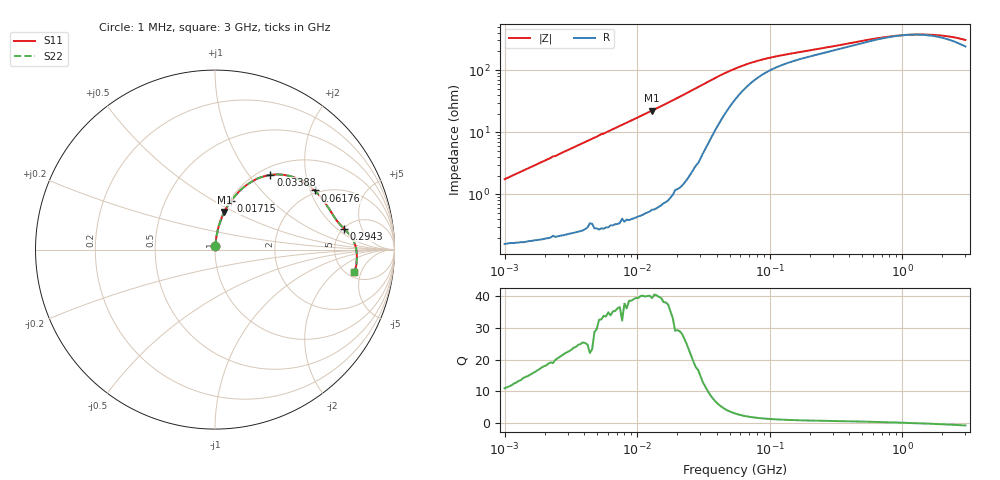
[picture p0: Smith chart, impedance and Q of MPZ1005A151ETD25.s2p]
! S-parameter Generated by TDK Corporation
! Copyright(C) 2018 TDK Corporation.
! All Rights Reserved.
! TDK P/N: MPZ1005A151ETD25 (Chip Bead)
! Property: |Z|=150¶ at 100MHz
! Size(LxWxT): 1x0.5x0.5mm, 0.039x0.02x0.02inches
! Model Type: s2p (Touchstone File Format Version 1.0)
! Frequency: DC=Yes Start=1MHz Stop=3000MHz 202points Log-sweep
! Model Generated on Aug. 6, 2018
! Port Assignments:
!  1 ---@@@--- 2
! Applicable Conditions:
!  Temperature = 25 degC
!  DC Bias Current = 0 A
!  Small Signal Operation
! Terms and conditions regarding TDK Simulation Models
! (1)This simulation model is being provided solely for informational purposes. Please refer to the specifications of the products in terms of detailed characteristics of such products.
! (2)In no event shall TDK Corporation of any of its subsidiaries be liable for any loss or damage arising, directly or indirectly,
!  From any information contained in this simulation model, including, but not limited to loss or damages arising from any inaccuracies, omissions or errors in connection with such information.
! (3)Any and all copyrights on this simulation model are owned by TDK Corporation.
!  Duplication or redistribution of this simulation model without prior written permission from TDK Corporation is prohibited.
! (4)This simulation model is subject to any modification or change without any prior notice.
! (5)Neither TDK Corporation nor any of its subsidiaries shall make any warranty, express or implied,
!  Including but not limited to the correctness, implied warranties of merchantability and fitness for a particular purpose with respect to this simulation models.
! (6)The use of this simulation model shall be deemed to have consented to the terms and conditions hereof.
# Hz S MA R 50
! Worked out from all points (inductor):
!   201 points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, 1 MHz to 3 GHz, reference 50 ohm
!   read as one part in series: L = 277 nH near 1.041 MHz
!   highest Q = 40.2 at 12.96 MHz (marker M1), where L = 274 nH
!   self-resonance near 1.124 GHz
!   S11 on the Smith chart (normalised r, x): 1 MHz: 1.00, +0.03; 17.15 MHz: 1.02, +0.60; 33.88 MHz: 1.12, +1.28; 61.76 MHz: 1.90, +2.15; 294.3 MHz: 5.06, +2.52; 3 GHz: 5.78, -3.81
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1000000  0.01749 83.8  0.9983 -1.0  0.9983 -1.0  0.01749 83.8
2317916  0.04067 84.6  0.997 -2.3  0.997 -2.3  0.04067 84.6
2412589  0.04125 84.8  0.9971 -2.4  0.9971 -2.4  0.04125 84.8
3900413  0.06662 83.9  0.9952 -3.8  0.9952 -3.8  0.06662 83.9
7703107  0.1296 80.8  0.9876 -7.4  0.9876 -7.4  0.1296 80.8
1.29622e7  0.2166 76.0  0.9708 -12.5  0.9708 -12.5  0.2166 76.0
1.461624e7  0.2433 74.5  0.9639 -14.1  0.9639 -14.1  0.2433 74.5
1.71545e7  0.2843 72.0  0.9512 -16.5  0.9512 -16.5  0.2843 72.0
2.459509e7  0.4002 64.0  0.8993 -23.6  0.8993 -23.6  0.4002 64.0
3.387922e7  0.5182 53.4  0.8066 -31.0  0.8066 -31.0  0.5182 53.4
4.307715e7  0.589 43.8  0.7045 -35.3  0.7045 -35.3  0.589 43.8
5.477226e7  0.6319 34.7  0.6 -36.8  0.6 -36.8  0.6319 34.7
6.176144e7  0.6453 30.7  0.5538 -36.5  0.5538 -36.5  0.6453 30.7
7.852918e7  0.6633 24.3  0.4801 -34.6  0.4801 -34.6  0.6633 24.3
1.081723e8  0.6788 18.3  0.4146 -31.0  0.4146 -31.0  0.6788 18.3
2.136344e8  0.71 11.4  0.3349 -24.8  0.3349 -24.8  0.71 11.4
2.942768e8  0.7281 9.3  0.3047 -22.6  0.3047 -22.6  0.7281 9.3
8.005644e8  0.7787 2.5  0.2247 -8.8  0.2247 -8.8  0.7787 2.5
1.147801e9  0.7877 -0.2  0.2123 0.6  0.2123 0.6  0.7877 -0.2
1.645649e9  0.7917 -3.1  0.2137 11.4  0.2137 11.4  0.7917 -3.1
2.266846e9  0.7917 -6.0  0.2284 21.4  0.2284 21.4  0.7917 -6.0
3e9  0.7859 -9.2  0.2572 29.3  0.2572 29.3  0.7859 -9.2
